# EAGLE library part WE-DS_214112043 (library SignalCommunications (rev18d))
WE-DS D-SUB-Filter Connectors Bent 90° Characteristics Standard type filtered with 1000 pF High attenuation of more than 40 dB @ 180 MHz Choice of earthing metal sheet or high speed earthing clip Rated voltage: 100 VDC Rated current @ 20 ºC: 5 A Withstand voltage: 250 VRMS Insulation resistance: min. 1000 MΩ Operating temperature: –55 ºC to +125 ºC Applications Filtering of interfaces External connection to -printer -sensor -display Details see: http://katalog.we-online.de/en/pbs/Filter_abgewinkelt Created on 2015-05-04 2015 (C) Wurth Elektronik
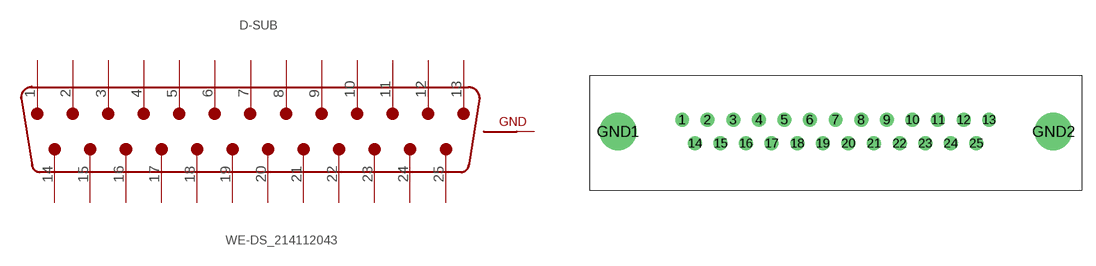
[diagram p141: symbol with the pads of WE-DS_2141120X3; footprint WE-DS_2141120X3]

Designator prefix D-SUB

## WE-DS_214112043 (WE-NUMBER: 214112043/25Pins_male)  [WE-DS_2141120X3]
1  1  pas
2  2  pas
3  3  pas
4  4  pas
5  5  pas
6  6  pas
7  7  pas
8  8  pas
9  9  pas
10  10  pas
11  11  pas
12  12  pas
13  13  pas
14  14  pas
15  15  pas
16  16  pas
17  17  pas
18  18  pas
19  19  pas
20  20  pas
21  21  pas
22  22  pas
23  23  pas
24  24  pas
25  25  pas
GND1  GND  pwr
GND2  GND  pwr

## Footprint WE-DS_2141120X3 (pad centres in mm)
drill 1: 1 -16.56,1.27; 2 -13.82,1.27; 3 -11.05,1.27; 4 -8.28,1.27; 5 -5.54,1.27; 6 -2.77,1.27; 7 0,1.27; 8 2.77,1.27; 9 5.54,1.27; 10 8.28,1.27; 11 11.05,1.27; 12 13.82,1.27; 13 16.56,1.27; 14 -15.19,-1.27; 15 -12.42,-1.27; 16 -9.68,-1.27; 17 -6.91,-1.27; 18 -4.14,-1.27; 19 -1.38,-1.27; 20 1.38,-1.27; 21 4.14,-1.27; 22 6.91,-1.27; 23 9.68,-1.27; 24 12.42,-1.27; 25 15.19,-1.27
drill 3: GND1 -23.5,0; GND2 23.5,0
